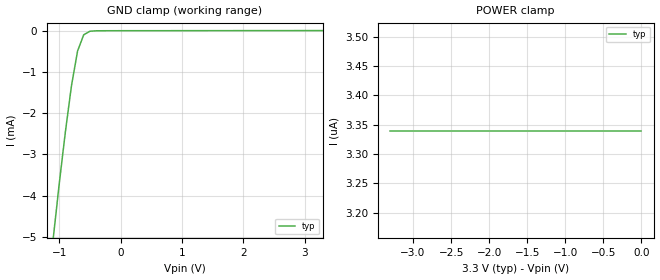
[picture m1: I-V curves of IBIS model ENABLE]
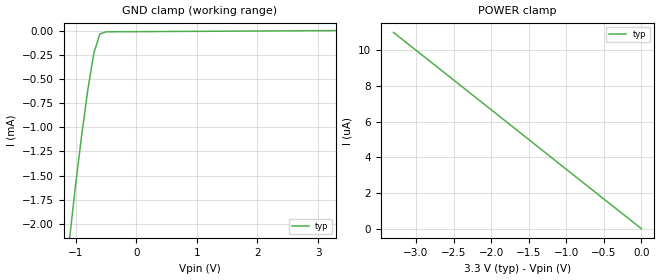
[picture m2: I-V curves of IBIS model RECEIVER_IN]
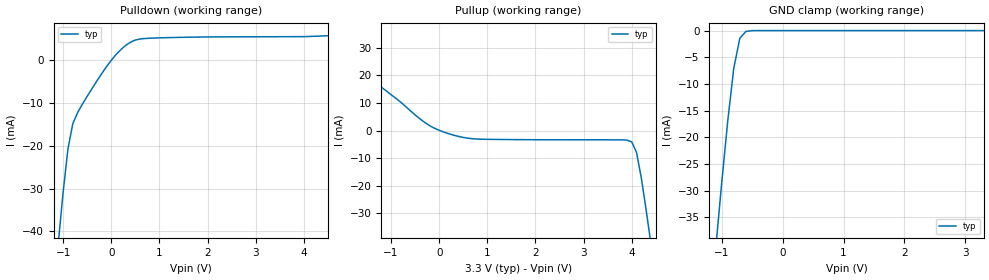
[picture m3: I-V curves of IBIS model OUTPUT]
|   Texas Instruments Incorporated
|   Data Transmissions Products
|   IBIS Model for SN65LVDS117
|   64DGG TSSOP Package
[IBIS Ver]   2.1
[Comment char]   |_char
[File name]   lvds117.ibs
[File Rev]   1.0
[Date]   17Jun99
[Source]   File originated at Texas Instruments Incorporated.
   Data Transmission Products Group.
[Notes]
[Disclaimer]
(C) Copyright Texas Instruments Incorporated 1999
   All rights reserved
  Texas Instruments Incorporated hereby grants the user of this IBIS
model a non-exclusive, nontransferable license to use this IBIS model
under the following terms.  Before using this IBIS model, the user
should read this license.  If the user does not accept these terms,
the IBIS model should be returned to Texas Instruments within 30 days.
  The user is granted this license only to use the IBIS model and
is not granted rights to sell, load, rent, lease or license the IBIS
model in whole or in part, or in modified form to anyone other than
user.  User may modify the IBIS model to suit its specific applications
but rights to derivative works and such modifications shall belong to
Texas Instruments.
  This IBIS model is provided on an "AS IS" basis and Texas Instruments
makes absolutely no warranty with respect to the information contained
herein.  TEXAS INSTRUMENTS DISCLAIMS AND CUSTOMER WAIVES ALL WARRANTIES,
EXPRESS OR IMPLIED, INCLUDING WARRANTIES OF MERCHANTABILITY OR FITNESS
FOR A PARTICULAR PURPOSE. The entire risk as to quality and performance
is with the Customer. ACCORDINGLY, IN NO EVENT SHALL THE COMPANY BE LIABLE
FOR ANY DAMAGES, WHETHER IN CONTRACT OR TORT,INCLUDING ANY LOST PROFITS
OR OTHER INCIDENTAL, CONSEQUENTIAL, EXEMPLARY, OR PUNITIVE DAMAGES ARISING
OUT OF THE USE OR APPLICATION OF THE IBIS model provided in this package.
Further, Texas Instruments reserves the right to discontinue or make changes
without notice to any product herein to improve reliability, function, or
design. Texas Instruments does not convey any license under patent rights
or any other intellectual property rights, including those of third parties.
Contact Texas Instruments at ATTN:DATA TRANSMISSIONS
Thomas Fisher 8505 Forest Lane, M/S 8710, Dallas, TX 75243-4136
[Copyright]   Copyright 1999, Texas Instruments, All Rights Reserved
[Component]   LVDS117DGG
[Manufacturer]  Texas Instruments Incorporated
[Package]
|   typ   min   max
R_pkg   0.068   0.046   0.094
L_pkg   3.798nH   2.565nH   5.991nH
C_pkg   0.564pF   0.297pF   1.022pF
[Pin]   signal_name   model_name   R_pin   L_pin   C_pin
1   GND   GND   0.094   5.991n   0.940p
2   VCC   POWER   0.090   5.514n   1.005p
3   VCC   POWER   0.092   5.261n   0.912p
4   GND   GND   0.092   4.891n   0.805p
5   NC   NC
6   ENM   ENABLE   0.084   4.247n   0.597p
7   ENA   ENABLE   0.080   3.933n   0.534p
8   ENB   ENABLE   0.077   3.622n   0.523p
9   ENC   ENABLE   0.050   3.372n   0.483p
10   END   ENABLE   0.048   3.139n   0.415p
11   NC   NC
12   GND   GND   0.051   2.941n   0.384p
13   1A   RECEIVER_IN   0.050   2.800n   0.355p
14   1B   RECEIVER_IN   0.052   2.711n   0.335p
15   GND   GND   0.051   2.589n   0.314p
16   VCC   POWER   0.055   2.604n   0.303p
17   VCC   POWER   0.055   2.597n   0.302p
18   GND   GND   0.052   2.605n   0.315p
19   2A   RECEIVER_IN   0.051   2.694n   0.334p
20   2B   RECEIVER_IN   0.050   2.772n   0.352p
21   GND   GND   0.048   2.864n   0.372p
22   NC   NC
23   ENE   ENABLE   0.049   3.129n   0.413p
24   ENF   ENABLE   0.046   3.263n   0.480p
25   ENG   ENABLE   0.077   3.592n   0.542p
26   ENH   ENABLE   0.081   3.923n   0.557p
27   NC   NC
28   NC   NC
29   GND   GND   0.087   4.810n   0.813p
30   VCC   POWER   0.089   5.135n   0.918p
31   VCC   POWER   0.090   5.486n   1.019p
32   GND   GND   0.090   5.912n   0.936p
33   H2Z   OUTPUT   0.087   5.926n   0.931p
34   H2Y   OUTPUT   0.087   5.496n   1.004p
35   H1Z   OUTPUT   0.087   5.124n   0.902p
36   H1Y   OUTPUT   0.088   4.867n   0.807p
37   G2Z   OUTPUT   0.086   4.514n   0.707p
38   G2Y   OUTPUT   0.085   4.206n   0.605p
39   G1Z   OUTPUT   0.089   3.929n   0.537p
40   G1Y   OUTPUT   0.079   3.584n   0.528p
41   F2Z   OUTPUT   0.048   3.299n   0.481p
42   F2Y   OUTPUT   0.048   3.101n   0.409p
43   F1Z   OUTPUT   0.048   2.969n   0.388p
44   F1Y   OUTPUT   0.048   2.855n   0.369p
45   E2Z   OUTPUT   0.049   2.766n   0.349p
46   E2Y   OUTPUT   0.051   2.696n   0.331p
47   E1Z   OUTPUT   0.052   2.638n   0.315p
48   E1Y   OUTPUT   0.053   2.565n   0.297p
49   D2Z   OUTPUT   0.052   2.574n   0.299p
50   D2Y   OUTPUT   0.051   2.617n   0.313p
51   D1Z   OUTPUT   0.050   2.666n   0.329p
52   D1Y   OUTPUT   0.050   2.769n   0.350p
53   C2Z   OUTPUT   0.049   2.909n   0.378p
54   C2Y   OUTPUT   0.048   2.993n   0.390p
55   C1Z   OUTPUT   0.049   3.176n   0.416p
56   C1Y   OUTPUT   0.048   3.295n   0.483p
57   B2Z   OUTPUT   0.079   3.569n   0.536p
58   B2Y   OUTPUT   0.082   3.908n   0.547p
59   B1Z   OUTPUT   0.086   4.238n   0.613p
60   B1Y   OUTPUT   0.086   4.509n   0.714p
61   A2Z   OUTPUT   0.089   4.863n   0.822p
62   A2Y   OUTPUT   0.090   5.197n   0.923p
63   A1Z   OUTPUT   0.092   5.558n   1.022p
64   A1Y   OUTPUT   0.090   5.947n   0.946p
[Diff_pin]   inv_pin   vdiff   tdelay_typ   tdelay_min   tdelay_max
| The 'xA' pin is Diff_pin and the 'xB' pin is the inv_pin
13   14   0.100   0 0 0
19   20   0.100   0 0 0
34   33   NA   0 0 0
36   35   NA   0 0 0
38   37   NA   0 0 0
40   39   NA   0 0 0
42   41   NA   0 0 0
44   43   NA   0 0 0
46   45   NA   0 0 0
48   47   NA   0 0 0
50   49   NA   0 0 0
52   51   NA   0 0 0
54   53   NA   0 0 0
56   55   NA   0 0 0
58   57   NA   0 0 0
60   59   NA   0 0 0
62   61   NA   0 0 0
64   63   NA   0 0 0
| Models and submodels in the file (3): ENABLE (Input), RECEIVER_IN (Input), OUTPUT (3-state)
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|   Enable Model
[Model]   ENABLE
Model_type   Input
|Signals   ENM,ENA,ENB,ENC,END,ENE,ENF,ENG,ENH
Vinh = 2.0
Vinl = 0.8
|   typ   min   max
C_comp   1.0pF   NA   NA
|   typ   min   max
[Temperature Range]   25.0   NA   NA
[Voltage range]   3.3V   3.0V   3.6V
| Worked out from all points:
|   GND clamp passes 1 mA (typ) near -0.76 V on its own axis
[GND_clamp]
|   Voltage   I(typ)   I(min)   I(max)
-3.3V     -43.1mA    NA         NA
-1.1V     -5.08mA    NA         NA
-1V       -3.73mA    NA         NA
-900mV    -2.47mA    NA         NA
-800mV    -1.34mA    NA         NA
-700mV    -493uA     NA         NA
-600mV    -98.5uA    NA         NA
-500mV    -13.3uA    NA         NA
3.3V      3.34uA     NA         NA
[Power_clamp]
| Note that the[POWER_clamp]voltage table is referenced to Vcc
| and is calculated using Vtable=Vcc - Vmeasured.
|   Voltage   I(typ)   I(min)   I(max)
-3.3V     3.34uA     NA         NA
-2.7V     3.34uA     NA         NA
-2V       3.34uA     NA         NA
-800mV    3.34uA     NA         NA
0V        3.34uA     NA         NA
|   Receiver Input MODEL
[Model]   RECEIVER_IN
Model_type   Input
|Signals   1A,1B,2A,2B
Vinh = 2.0
Vinl = 0.8
|   typ   min   max
C_comp   1.0pF   NA   NA
|   typ   min   max
[Temperature Range]   25.0   NA   NA
[Voltage range]   3.3V   3.0V   3.6V
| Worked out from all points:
|   GND clamp passes 1 mA (typ) near -0.88 V on its own axis
[GND_clamp]
|   Voltage   I(typ)   I(min)   I(max)
-3.3V     -22.5mA    NA         NA
-1.1V     -2.15mA    NA         NA
-1V       -1.59mA    NA         NA
-900mV    -1.08mA    NA         NA
-800mV    -616uA     NA         NA
-700mV    -234uA     NA         NA
-600mV    -34.5uA    NA         NA
-500mV    -13.2uA    NA         NA
-400mV    -12.3uA    NA         NA
3.3V      444pA      NA         NA
[Power_clamp]
| Note that the[POWER_clamp]voltage table is referenced to Vcc
| and is calculated using Vtable=Vcc - Vmeasured.
|   Voltage   I(typ)   I(min)   I(max)
-3.3V     11uA       NA         NA
-2V       6.67uA     NA         NA
-1V       3.33uA     NA         NA
0V        0A         NA         NA
|   Driver Output  MODEL
[Model]   OUTPUT
Model_type   3-state
| Signals   A1Y,A1Z,A2Y,A2Z,B1Y,B1Z,B2Y,B2Z,C1Y,C1Z,C2Y,C2Z,D1Y,D1Z,D2Y,D2Z,
|   E1Y,E1Z,E2Y,E2Z,F1Y,F1Z,F2Y,F2Z,G1Y,G1Z,G2Y,G2Z,H1Y,H1Z,H2Y,H2Z
Vmeas = 1.2V   |Reference voltage for timing measurements
Cref = 5pF   |Timing specification test load capacitance value
Rref = 50   |Note: 50 Ohm load; single ended configuration
Vref = 1.18V   |Timing specification test load voltage
| variable   typ   min   max
C_comp   1.0pF   NA   NA
|   typ   min   max
[Temperature Range]   25.0   NA   NA
[Voltage range]   3.3V   3.0V   3.6V
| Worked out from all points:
|   slope of the pulldown table from 0 to 0.495 V, typ, clamps not added: 105 ohm
|   slope of the pullup table from 0 to 0.495 V, typ, clamps not added: 192 ohm
|   GND clamp passes 1 mA (typ) near -0.67 V on its own axis
[Pulldown]
|   Voltage   I(typ)   I(min)   I(max)
-3.3V     -348mA     NA         NA
-1.1V     -42.6mA    NA         NA
-1V       -30.8mA    NA         NA
-900mV    -20.7mA    NA         NA
-800mV    -14.9mA    NA         NA
-600mV    -10.3mA    NA         NA
-100mV    -1.58mA    NA         NA
200mV     2.42mA     NA         NA
500mV     4.64mA     NA         NA
1.4V      5.26mA     NA         NA
4.1V      5.46mA     NA         NA
6.6V      7.11mA     NA         NA
[Pullup]
|   Voltage   I(typ)   I(min)   I(max)
| Note that the[Pullup]voltage table is referenced to Vcc
| and is calculated using Vtable=Vcc - Vmeasured.
-3.3V     49.3mA     NA         NA
-2.6V     37.7mA     NA         NA
-1.9V     25.6mA     NA         NA
-400mV    4.24mA     NA         NA
200mV     -1.17mA    NA         NA
800mV     -3.11mA    NA         NA
4V        -4.13mA    NA         NA
4.1V      -8.04mA    NA         NA
4.2V      -17.4mA    NA         NA
4.3V      -29mA      NA         NA
4.4V      -41.4mA    NA         NA
6.6V      -348mA     NA         NA
[GND_clamp]
|   Voltage   I(typ)   I(min)   I(max)
| Outputs in High Impedance (off)
-3.3V     -347mA     NA         NA
-1.1V     -41.4mA    NA         NA
-1V       -28.8mA    NA         NA
-900mV    -17.1mA    NA         NA
-800mV    -7.08mA    NA         NA
-700mV    -1.43mA    NA         NA
-600mV    -153uA     NA         NA
-400mV    -866nA     NA         NA
3.3V      -59.7pA    NA         NA
[POWER_clamp]
|   Voltage   I(typ)   I(min)   I(max)
| Note that the [POWER_clamp] voltage table is referenced to Vcc
| and is calculated using Vtable = Vcc - Vmeasured.
| Outputs in Tri-state.
-3.3V     0A         NA         NA
0V        0A         NA         NA
[Ramp]
|   typ   min   max
dV/dt_r   0.346/600ps   NA   NA
dV/dt_f   0.309/600ps   NA   NA
R_load = 100ohm | Note: The measurement is on a differential configuration
